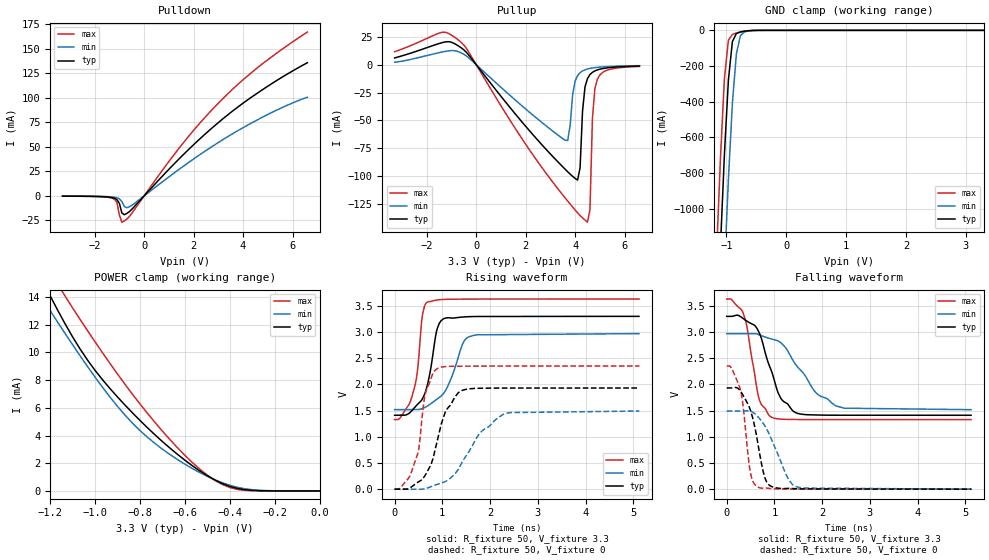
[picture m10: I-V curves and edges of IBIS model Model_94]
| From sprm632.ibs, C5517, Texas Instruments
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| Model based on original model for BC3340CTSCHYPD
|   Sub model SR0_VSS_SR1_VSS_PD_OFF_IND_3P3
[model]   Model_94
|[Description]  [3.3V-I/O-PD_OFF-X, IND]
|   PD_OFF,IND,
|[Input Load]   PD_OFF
|[Output Drive]
|Voltage   3.3V
|Mode   I/O
Model_type   I/O
Polarity   Non-Inverting
Enable   Active-Low
Vinl =  0.8
Vinh =  2
Cref =  15.0000pF
Rref =  100.0000M
Vref =  0V
Vmeas =  1.65
C_comp   2.113745p   2.0494201p   2.2478119p
[Model Spec]
Vinl   0.8   0.8   0.8
Vinh   2   2   2
[Temperature Range]   25   105   -40
[Voltage Range]   3.3   2.97   3.63
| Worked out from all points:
|   slope of the pulldown table from 0 to 0.495 V, typ, clamps not added: 36.4 ohm
|   slope of the pullup table from 0 to 0.495 V, typ, clamps not added: 34.9 ohm
|   GND clamp passes 1 mA (typ) near -0.57 V on its own axis
|   POWER clamp passes 1 mA (typ) near -0.49 V on its own axis
|   rising waveform, R_fixture 50, V_fixture 3.3: 20-80 % time 244ps typ, 379ps min, 193ps max; typ from 1.41 V to 3.3 V
|   rising waveform, R_fixture 50, V_fixture 0: 20-80 % time 397ps typ, 707ps min, 257ps max; typ from 0 V to 1.93 V
|   falling waveform, R_fixture 50, V_fixture 3.3: 20-80 % time 394ps typ, 661ps min, 254ps max; typ from 3.3 V to 1.41 V
|   falling waveform, R_fixture 50, V_fixture 0: 20-80 % time 271ps typ, 424ps min, 180ps max; typ from 1.93 V to 0 V
[POWER_clamp]
-3.3V     86.08mA    66.79mA    104.2mA
-1.267V   16.23mA    14.68mA    17.92mA
-1.233V   15.14mA    13.84mA    16.84mA
-1.2V     14.07mA    13mA       15.85mA
-1.133V   12.04mA    11.35mA    14.05mA
-1V       8.692mA    8.203mA    10.75mA
-833.3mV  5.628mA    4.887mA    6.97mA
-666.7mV  3.091mA    2.627mA    3.701mA
-500mV    1.094mA    1.049mA    1.134mA
-433.3mV  532.4uA    589.2uA    463.5uA
-366.7mV  181.3uA    262.8uA    110.8uA
0V        865.7pA    6.551nA    589.7pA
[Pulldown]
-3.3V     -240.7uA   -180.9uA   -268.6uA
-1.3V     -1.697mA   -1.064mA   -2.248mA
-1.1V     -3.762mA   -1.923mA   -6.664mA
-1V       -7.728mA   -3.048mA   -19.72mA
-900mV    -17.44mA   -5.882mA   -26.83mA
-800mV    -19.19mA   -10.95mA   -25.48mA
-700mV    -17.88mA   -12.05mA   -23.65mA
-500mV    -13.74mA   -9.678mA   -17.88mA
1.5V      39.94mA    28.65mA    51.42mA
2.9V      72.6mA     52.84mA    91.93mA
4.6V      105.1mA    77.82mA    131.1mA
6.6V      135.8mA    100.6mA    167.1mA
[Pullup]
-3.3V     6.015mA    2.203mA    11.63mA
-700mV    16.55mA    11.47mA    21.8mA
3.6V      -93.97mA   -67.88mA   -119.8mA
3.7V      -96.18mA   -68.06mA   -122.5mA
4.1V      -103.6mA   -9.75mA    -133mA
4.2V      -92.66mA   -7.165mA   -135.5mA
4.3V      -41.55mA   -5.629mA   -137.6mA
4.5V      -12.4mA    -3.913mA   -141.5mA
4.6V      -8.869mA   -3.389mA   -130.3mA
4.7V      -6.864mA   -2.987mA   -48.17mA
4.9V      -4.698mA   -2.411mA   -13mA
6.6V      -1.25mA    -906.2uA   -1.586mA
[GND_clamp]
-3.3V     -22.46A    -23.08A    -22.02A
-1.167V   -1.78A     -2.475A    -1.268A
-1.1V     -1.214A    -1.896A    -719.3mA
-1.033V   -694.9mA   -1.343A    -269mA
-966.7mV  -277.7mA   -834.1mA   -54.76mA
-900mV    -62.9mA    -407mA     -23.12mA
-833.3mV  -17.79mA   -131.4mA   -15.05mA
-766.7mV  -9.259mA   -30.27mA   -9.03mA
-700mV    -5.097mA   -8.689mA   -4.435mA
-433.3mV  -45.78uA   -150.7uA   -10.52uA
3.3V      865.7pA    147.8uA    436.6pA
[Ramp]
dV/dt_f  1.1472472/0.39640381n 0.88264168/0.66764337n  1.3953577/0.25805004n
dV/dt_r  1.1611302/0.39535143n  0.8971165/0.7072549n  1.4124725/0.25787378n
R_load = 50
[Rising Waveform]
R_fixture = 50
V_fixture = 3.3
V_fixture_min = 2.97
V_fixture_max = 3.63
0s        1.411V     1.519V     1.329V
368.7ps   1.506V     1.521V     1.785V
474.6ps   1.613V     1.521V     2.231V
588.8ps   1.735V     1.542V     3.356V
686.2ps   1.989V     1.587V     3.571V
888.4ps   3.05V      1.719V     3.611V
1.045ns   3.261V     1.852V     3.624V
1.427ns   3.287V     2.776V     3.629V
1.642ns   3.296V     2.934V     3.629V
5.12ns    3.3V       2.97V      3.63V
[Rising Waveform]
R_fixture = 50
V_fixture = 0
V_fixture_min = 0
V_fixture_max = 0
0s        0V         0V         0V
344.6ps   37.65mV    0V         305.8mV
506.8ps   143.1mV    0V         767.6mV
656.3ps   289.7mV    14.29mV    1.862V
900.3ps   948.6mV    94.26mV    2.305V
1.067ns   1.486V     146.2mV    2.341V
1.335ns   1.842V     377.2mV    2.348V
1.767ns   1.926V     1.047V     2.35V
2.264ns   1.93V      1.424V     2.35V
5.129ns   1.931V     1.492V     2.351V
[Falling Waveform]
R_fixture = 50
V_fixture = 3.3
V_fixture_min = 2.97
V_fixture_max = 3.63
0s        3.299V     2.969V     3.63V
340.6ps   3.261V     2.969V     3.371V
433.9ps   3.202V     2.969V     3.054V
680.4ps   2.987V     2.947V     1.719V
943.8ps   2.241V     2.865V     1.373V
1.136ns   1.731V     2.794V     1.337V
1.412ns   1.477V     2.425V     1.33V
1.883ns   1.416V     1.83V      1.329V
2.29ns    1.412V     1.589V     1.328V
5.12ns    1.411V     1.518V     1.328V
[Falling Waveform]
R_fixture = 50
V_fixture = 0
V_fixture_min = 0
V_fixture_max = 0
0s        1.932V     1.491V     2.351V
93.3ps    1.932V     1.491V     2.32V
291.2ps   1.868V     1.491V     1.883V
490.2ps   1.526V     1.491V     354.7mV
643.8ps   923.8mV    1.392V     43.75mV
760.5ps   352.3mV    1.262V     18.62mV
882.8ps   84.2mV     1.068V     15.61mV
1.282ns   14.69mV    209.6mV    2.481mV
1.486ns   6.983mV    37.67mV    1.495mV
5.129ns   538.2nV    66uV       0V
